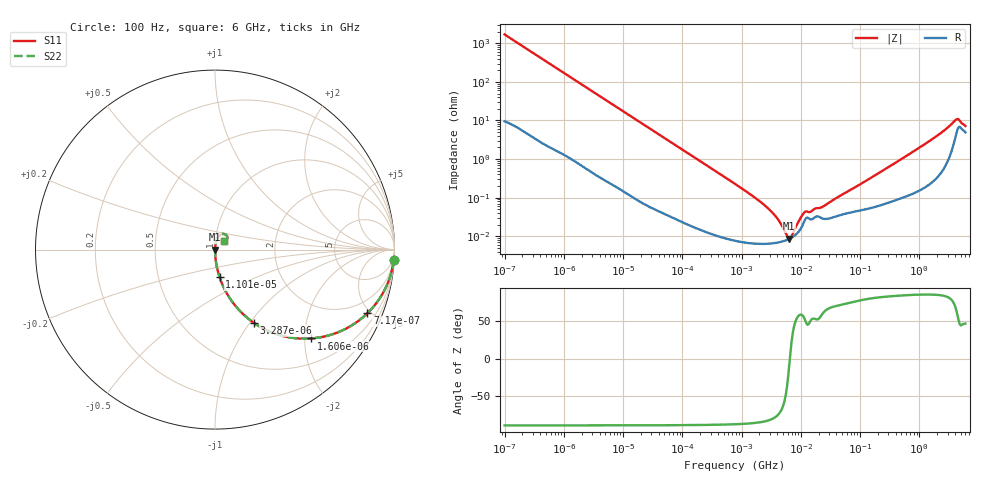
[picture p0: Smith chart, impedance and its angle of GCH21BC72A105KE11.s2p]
!Murata Part Number: GCH21BC72A105KE11
!These Parameters are Measured in Series Mode Connection
!Data Generated on Jun 19, 2026
!  o--ll--o
!Port1  Port2
!  o------o
!Operation Temp=25[degC], DC Bias Voltage=0[V]
!Freq. Start=100[Hz] Stop=6[GHz] 401[Steps]
# Hz S RI R 50
!Freq.(Hz) S11(Real) S11(Imag) S21(Real) S21(Imag) S12(Real) S12(Imag) S22(Real) S22(Imag)
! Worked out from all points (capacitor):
!   401 points, 100 Hz to 6 GHz, reference 50 ohm
!   read as one part in series: C = 936 nF near 109 Hz
!   lowest |Z| = 8.62 mohm at 6.353 MHz (marker M1)
!   series resonance near 6.531 MHz, so ESL is about 630 pH
!   S11 on the Smith chart (normalised r, x): 100 Hz: 1, -34; 717 Hz: 1.03, -4.78; 1.606 kHz: 1.02, -2.14; 3.287 kHz: 1.01, -1.05; 11.01 kHz: 1.00, -0.32; 6 GHz: 1.10, +0.10
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100  0.9962 -0.0587  0.00378 0.0587  0.00378 0.0587  0.9962 -0.0587
335  0.9618 -0.1885  0.0382 0.1885  0.0382 0.1885  0.9618 -0.1885
717  0.849 -0.3545  0.151 0.3545  0.151 0.3545  0.849 -0.3545
1606  0.5341 -0.495  0.4659 0.495  0.4659 0.495  0.5341 -0.495
2008  0.4242 -0.4904  0.5758 0.4904  0.5758 0.4904  0.4242 -0.4904
3287  0.2179 -0.409  0.7821 0.409  0.7821 0.409  0.2179 -0.409
5625  0.0883 -0.2797  0.9117 0.2797  0.9117 0.2797  0.0883 -0.2797
11009  0.0255 -0.1535  0.9745 0.1535  0.9745 0.1535  0.0255 -0.1535
40335  0.00231 -0.0432  0.9977 0.0432  0.9977 0.0432  0.00231 -0.0432
774597  8.11e-05 -0.00227  0.9999 0.00227  0.9999 0.00227  8.11e-05 -0.00227
2967816  6.43e-05 -0.000481  0.9999 0.000481  0.9999 0.000481  6.43e-05 -0.000481
4060267  6.83e-05 -0.000273  0.9999 0.000273  0.9999 0.000273  6.83e-05 -0.000273
6353432  8.48e-05 -1.54e-05  0.9999 1.54e-05  0.9999 1.54e-05  8.48e-05 -1.54e-05
7266822  9.51e-05 6.1e-05  0.9999 -6.1e-05  0.9999 -6.1e-05  9.51e-05 6.1e-05
1.137099e7  0.000236 0.000332  0.9998 -0.000332  0.9998 -0.000332  0.000236 0.000332
1.555665e7  0.000276 0.000368  0.9997 -0.000368  0.9997 -0.000368  0.000276 0.000368
2.434276e7  0.000282 0.000529  0.9997 -0.000529  0.9997 -0.000529  0.000282 0.000529
3.124326e8  0.000791 0.00634  0.9992 -0.00634  0.9992 -0.00634  0.000791 0.00634
1.791126e9  0.00404 0.0354  0.996 -0.0354  0.996 -0.0354  0.00404 0.0354
4.009986e9  0.0404 0.0872  0.9596 -0.0872  0.9596 -0.0872  0.0404 0.0872
4.586474e9  0.068 0.0739  0.932 -0.0739  0.932 -0.0739  0.068 0.0739
6e9  0.0492 0.0476  0.9508 -0.0476  0.9508 -0.0476  0.0492 0.0476
